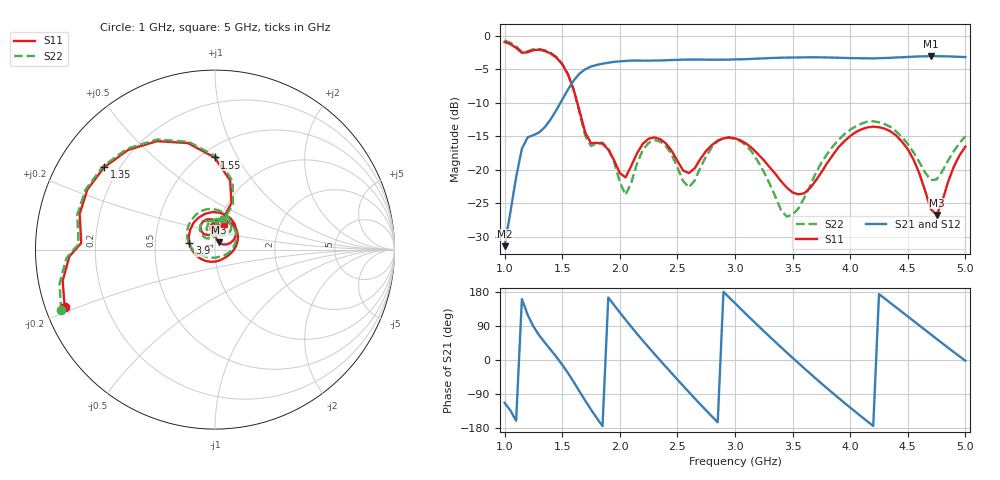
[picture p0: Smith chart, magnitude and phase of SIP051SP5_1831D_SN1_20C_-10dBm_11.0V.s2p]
# GHz  S  dB  R  50
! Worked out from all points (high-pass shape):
!   81 points, 1 GHz to 5 GHz, reference 50 ohm
!   highest |S21| = -3.05 dB at 4.7 GHz (marker M1); lowest = -31.4 dB at 1 GHz (marker M2)
!   |S21| within 3 dB of the highest: 1.631 GHz to end of sweep
!   lowest |S11| = -26.7 dB at 4.75 GHz (marker M3), VSWR 1.10, Z = 52.1 + j4.2 ohm
!   |S11| at or under -10 dB: 1.631 GHz to end of sweep
!   |S22| runs from -27.0 to -0.7 dB; largest |S21 - S12| = 0.0023
!   S11 on the Smith chart (normalised r, x): 1 GHz: 0.06, -0.18; 1.35 GHz: 0.14, +0.32; 1.55 GHz: 0.58, +0.81; 3.9 GHz: 0.75, +0.05; 5 GHz: 1.06, +0.30
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1  -0.95 -159.0  -31.41 -113.0  -31.52 -113.4  -0.71 -158.4
1.15  -2.54 177.2  -16.87 160.6  -16.89 160.7  -2.37 177.8
1.35  -2.28 143.3  -13.63 45.5  -13.63 45.4  -2.18 143.4
1.55  -5.79 90.3  -8.03 -34.3  -8.01 -34.3  -5.75 89.0
1.7  -14.46 74.6  -5.00 -107.3  -5.01 -107.3  -14.95 73.8
1.85  -16.13 93.2  -4.18 -174.5  -4.17 -174.5  -15.95 92.5
2.05  -21.14 113.7  -3.77 106.3  -3.77 106.2  -23.75 107.5
2.2  -16.12 121.6  -3.72 51.0  -3.73 51.0  -17.04 127.4
2.35  -15.43 95.5  -3.69 -0.9  -3.70 -1.0  -15.79 98.6
2.5  -18.69 79.7  -3.61 -51.5  -3.60 -51.5  -19.65 77.9
2.65  -19.78 100.1  -3.56 -101.1  -3.56 -101.0  -21.62 108.3
2.85  -15.66 84.6  -3.58 -164.5  -3.60 -164.5  -15.73 95.5
3  -15.31 56.5  -3.54 149.9  -3.54 149.8  -15.40 63.3
3.3  -19.61 -0.7  -3.33 61.9  -3.34 61.9  -22.06 -12.6
3.5  -23.40 -50.5  -3.26 5.7  -3.25 5.7  -26.68 -99.6
3.7  -21.65 -130.3  -3.22 -48.6  -3.23 -48.5  -20.54 -164.3
3.9  -16.62 166.2  -3.29 -100.4  -3.29 -100.6  -15.53 157.4
4.15  -13.68 105.3  -3.37 -162.2  -3.38 -162.1  -12.82 110.2
4.35  -14.27 62.6  -3.30 150.4  -3.30 150.3  -13.61 75.2
4.7  -25.87 35.6  -3.05 67.6  -3.05 67.7  -21.56 67.2
4.75  -26.74 61.0  -3.06 55.7  -3.05 55.8  -21.45 79.1
5  -16.56 70.8  -3.19 -2.1  -3.19 -2.1  -15.00 74.9
